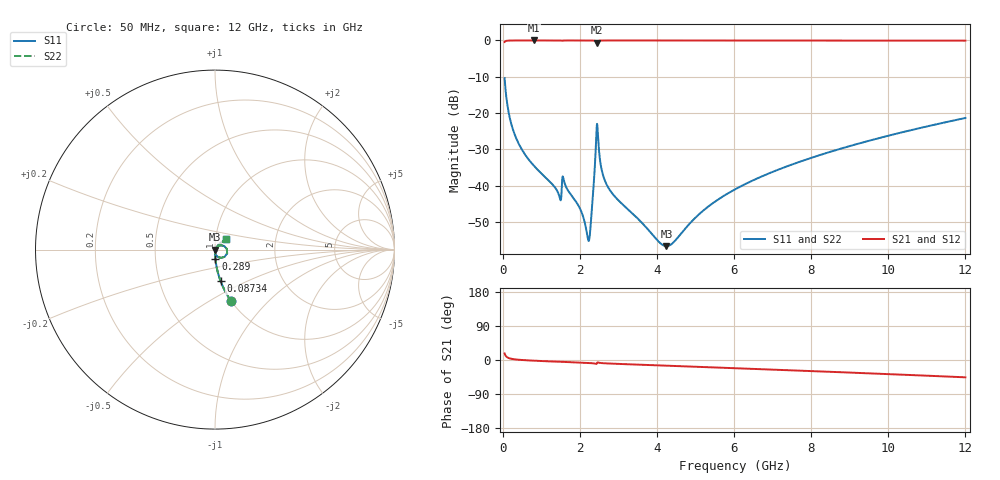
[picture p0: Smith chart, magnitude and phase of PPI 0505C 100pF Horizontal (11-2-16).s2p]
# MHz S MA R 50
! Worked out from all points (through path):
!   1601 points, 50 MHz to 12 GHz, reference 50 ohm
!   highest |S21| = -0.01 dB at 819.3 MHz (marker M1); lowest = -0.6 dB at 2.447 GHz (marker M2)
!   group delay of S21, straight-line fit = 10.9 ps
!   lowest |S11| = -56.7 dB at 4.247 GHz (marker M3), VSWR 1.00, Z = 50.1 - j0.0437 ohm
!   |S11| at or under -10 dB: start of sweep to end of sweep
!   |S22| runs from -56.7 to -10.4 dB; largest |S21 - S12| = 0
!   S11 on the Smith chart (normalised r, x): 50 MHz: 1.00, -0.63; 87.34 MHz: 1.00, -0.36; 289 MHz: 1.00, -0.11; 12 GHz: 1.13, +0.13
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50  0.3023 -72.5  0.953 17.4  0.953 17.4  0.3023 -72.5
87.34375  0.1786 -79.9  0.9836 10.0  0.9836 10.0  0.1786 -79.9
169.5  0.093 -85.0  0.9953 4.7  0.9953 4.7  0.093 -85.0
289  0.05453 -87.4  0.998 2.1  0.998 2.1  0.05453 -87.4
819.2812  0.01852 -89.6  0.999 -1.9  0.999 -1.9  0.01852 -89.6
1461.594  0.007353 -82.5  0.9983 -4.8  0.9983 -4.8  0.007353 -82.5
1603.5  0.01092 -83.8  0.9977 -5.1  0.9977 -5.1  0.01092 -83.8
2044.156  0.004318 -80.1  0.9986 -7.0  0.9986 -7.0  0.004318 -80.1
2193.531  0.002053 -49.2  0.9983 -7.7  0.9983 -7.7  0.002053 -49.2
2245.812  0.001816 0.9  0.9981 -8.0  0.9981 -8.0  0.001816 0.9
2305.562  0.004177 45.4  0.9974 -8.4  0.9974 -8.4  0.004177 45.4
2410.125  0.0294 45.0  0.9827 -9.9  0.9827 -9.9  0.0294 45.0
2447.469  0.0709 -17.6  0.9299 -8.0  0.9299 -8.0  0.0709 -17.6
2484.812  0.03703 -73.9  0.9848 -6.9  0.9848 -6.9  0.03703 -73.9
2596.844  0.01427 -89.6  0.9975 -8.4  0.9975 -8.4  0.01427 -89.6
2761.156  0.008962 -90.2  0.9984 -9.3  0.9984 -9.3  0.008962 -90.2
4038.312  0.001705 -47.4  0.9983 -14.2  0.9983 -14.2  0.001705 -47.4
4247.438  0.001462 -17.4  0.9983 -15.0  0.9983 -15.0  0.001462 -17.4
6025  0.008861 56.9  0.9978 -21.7  0.9978 -21.7  0.008861 56.9
8019.156  0.02426 55.7  0.9971 -29.3  0.9971 -29.3  0.02426 55.7
10013.31  0.04881 49.8  0.9957 -37.3  0.9957 -37.3  0.04881 49.8
12000  0.08537 42.3  0.9926 -45.7  0.9926 -45.7  0.08537 42.3
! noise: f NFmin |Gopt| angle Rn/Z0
50  0.0003582  0.8537  0.4061  0.0005224
1372  0.003852  0.6648  4.923  0.002199
2701  0.006541  0.6225  9.65  0.003215
4031  0.007818  0.5518  14.26  0.003072
5360  0.009704  0.5301  18.81  0.00355
6682  0.01154  0.5164  23.23  0.004013
8012  0.01338  0.5081  27.55  0.004482
9341  0.01524  0.5043  31.73  0.00497
1.067e+04  0.01716  0.5043  35.76  0.00549
1.2e+04  0.01916  0.5075  39.63  0.006058
